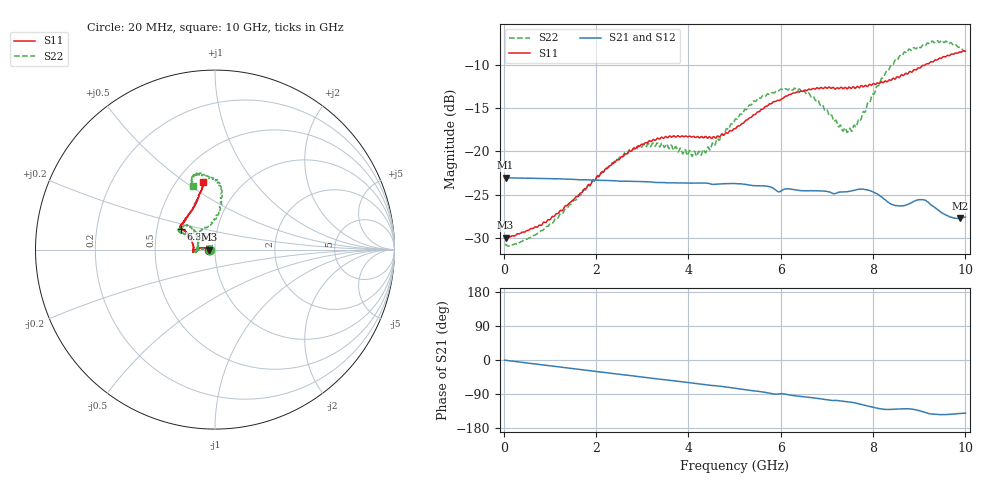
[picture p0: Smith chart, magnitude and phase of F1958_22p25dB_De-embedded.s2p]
! Integrated Device Technology
! Corporate Headquarters
! 6024 Silver Creek Valley Road
! San Jose, CA 95138  USA
! Phone:  1-408-284-8200
! Toll Free:  1-800-223-1366
! Webpage:  http://www.idt.com/
! Timing and RF Division
! 515 Groton Road, Suite 102
! Westford, MA 01886-6024
! Device:  F1958
! Description: 7-bit 0.25 dB Digital Step Attenuator
! Frequency:  0.001 -  6.000 GHz
! Package:  4x4 mm Thin QFN Plastic Package: 24 pin
! Ports:  2 RF, 12 DC
!  Pin  1  = D0
!  Pin  2  = VDD
!  Pin  3  = VMODE
!  Pin  4  = GND
!  Pin  5  = RF1  =  Port 1
!  Pin  6  = GND
!  Pin  7  = GND
!  Pin  8  = GND
!  Pin  9  = GND
!  Pin 10  = GND
!  Pin 11  = GND
!  Pin 12  = GND
!  Pin 13  = GND
!  Pin 14  = RF2  =  Port 2
!  Pin 15  = GND
!  Pin 16  = LE
!  Pin 17  = CLK
!  Pin 18  = DATA
!  Pin 19  = D6
!  Pin 20  = D5
!  Pin 21  = D4
!  Pin 22  = D3
!  Pin 23  = D2
!  Pin 24  = D1
! State:  89
! Atten State:  22.25 dB
! Voltage:  +3.30 Volts
! Current:  0.258 mA
! Data:  The device was measured on a F1958 evaluation board which has
!  individual transmission lines to the RF pins.  Data was collected
!  using a calibrated network analyzer.  The evaluation board was
!  de-embedded using Automatic Fixture Removal (AFR).
!  The reference plane is the edge of the package pin.
! Misc:
!  Action Tracker AT0419
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# GHz S dB R 50
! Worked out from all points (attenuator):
!   500 points, 20 MHz to 10 GHz, reference 50 ohm
!   highest |S21| = -23.06 dB at 40 MHz (marker M1); lowest = -27.8 dB at 9.88 GHz (marker M2)
!   lowest |S11| = -30.0 dB at 40 MHz (marker M3), VSWR 1.07, Z = 46.9 - j0.0415 ohm
!   |S11| at or under -10 dB: start of sweep to 9.13 GHz
!   |S22| runs from -31.0 to -7.2 dB; largest |S21 - S12| = 0.00032
!   S11 on the Smith chart (normalised r, x): 20 MHz: 0.94, -0.00; 6.36 GHz: 0.67, +0.16; 10 GHz: 0.67, +0.59
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0.02  -29.97 -178.9  -23.06 -0.4  -23.06 -0.3  -30.83 -178.8
0.04  -30.00 -179.2  -23.06 -0.7  -23.06 -0.7  -30.78 -178.2
0.84  -28.40 171.0  -23.14 -12.9  -23.13 -12.9  -29.16 176.4
1.7  -24.76 171.1  -23.29 -25.7  -23.29 -25.7  -24.71 175.1
2.62  -20.36 177.2  -23.45 -39.3  -23.43 -39.3  -20.15 -178.7
3.36  -18.56 -175.6  -23.61 -50.4  -23.60 -50.5  -19.33 -171.6
4.24  -18.45 -178.9  -23.67 -63.0  -23.68 -63.0  -20.02 166.6
4.64  -18.21 171.9  -23.79 -68.5  -23.80 -68.6  -18.53 148.6
5.02  -17.37 160.9  -23.73 -74.7  -23.74 -74.7  -16.24 138.2
5.58  -15.13 150.7  -23.99 -83.8  -24.01 -83.8  -13.78 138.6
6.36  -13.12 148.2  -24.48 -95.2  -24.50 -95.1  -13.01 151.8
6.68  -12.78 146.7  -24.56 -99.4  -24.57 -99.3  -13.67 152.8
7.3  -12.58 140.9  -24.71 -108.1  -24.71 -108.0  -16.97 132.1
7.5  -12.60 138.3  -24.62 -111.1  -24.62 -110.9  -17.32 114.0
7.68  -12.56 135.4  -24.39 -115.1  -24.39 -115.0  -16.36 97.1
7.9  -12.37 129.0  -24.48 -121.9  -24.48 -121.9  -14.36 88.1
8.34  -11.75 119.1  -25.92 -130.6  -25.92 -130.7  -10.62 82.5
8.7  -10.97 112.5  -26.25 -128.7  -26.23 -128.6  -8.53 88.0
9.06  -10.10 106.9  -25.59 -135.9  -25.62 -135.7  -7.81 94.8
9.26  -9.62 104.8  -26.22 -142.4  -26.23 -142.5  -7.37 99.6
9.88  -8.50 100.2  -27.77 -141.1  -27.76 -141.1  -7.95 108.4
10  -8.40 99.8  -27.61 -140.4  -27.62 -140.3  -8.47 108.9
